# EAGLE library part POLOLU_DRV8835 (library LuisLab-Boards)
Pololu DRV8835 Dual Motor Driver Carrier
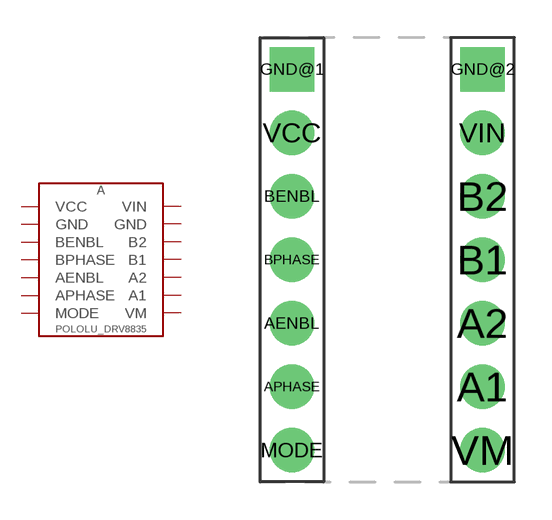
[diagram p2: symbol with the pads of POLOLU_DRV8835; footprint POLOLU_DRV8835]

Designator prefix A

## POLOLU_DRV8835  [POLOLU_DRV8835]
A1  A1
A2  A2
AENBL  AENBL
APHASE  APHASE
B1  B1
B2  B2
BENBL  BENBL
BPHASE  BPHASE
GND@1  GND
GND@2  GND
MODE  MODE
VCC  VCC
VIN  VIN
VM  VM

## Footprint POLOLU_DRV8835 (pad centres in mm)
Pololu DRV8835 Dual Motor Driver Carrier [Product Page] This tiny breakout board for TI’s DRV8835 dual motor driver can deliver 1.2 A per channel continuously (1.5 A peak) to a pair of DC motors, and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
drill 1 pad 1.778: A1 3.81,-5.08; A2 3.81,-2.54; AENBL -3.81,-2.54; APHASE -3.81,-5.08; B1 3.81,0; B2 3.81,2.54; BENBL -3.81,2.54; BPHASE -3.81,0; MODE -3.81,-7.62; VCC -3.81,5.08; VIN 3.81,5.08; VM 3.81,-7.62
drill 1 pad 1.778 square: GND@1 -3.81,7.62; GND@2 3.81,7.62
